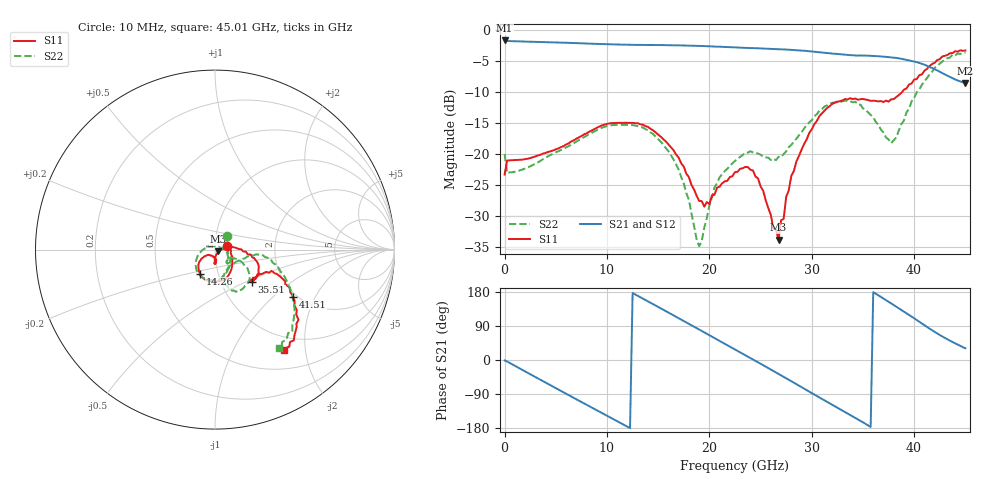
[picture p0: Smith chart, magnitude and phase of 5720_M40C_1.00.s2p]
! Device:  ADRF5720
! Description: 0.5dB LSB GaAs MMIC 6-bit Digital Attenuator
! Frequency:  0.000009 -  40 GHz
! Ports:
!	RF1	= Port 1
!	RF2	= Port 2
! Vdd:  3.3 Volt
! Vss:  -3.3 Volt
! Control:  0/3.3 Volt
! State:  1.00 dB attenuation
! Data:  The device was measured using G-S-G Probes on a matrix board.
!  Data was collected using an calibrated 4 port network analyzer.
!  The reference plane for this measurement is at the launchers.
! Note:  Analog Devices supplies this data as a sample of measured data
!  for this product.  Your particular data for this product may vary.
!  Data was taken at -40 degrees C.
!  Analog Devices reserves the right to change this data at anytime.
# GHZ S DB R 45.0
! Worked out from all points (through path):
!   181 points, 10 MHz to 45.01 GHz, reference 45 ohm
!   highest |S21| = -1.76 dB at 10 MHz (marker M1); lowest = -8.6 dB at 45.01 GHz (marker M2)
!   group delay of S21, straight-line fit = 42.4 ps
!   lowest |S11| = -33.8 dB at 26.76 GHz (marker M3), VSWR 1.04, Z = 46.6 - j0.912 ohm
!   |S11| at or under -10 dB: start of sweep to 38.85 GHz
!   |S22| runs from -34.9 to -3.7 dB; largest |S21 - S12| = 0.0032
!   S11 on the Smith chart (normalised r, x): 10 MHz: 1.14, +0.05; 14.26 GHz: 0.82, -0.23; 35.51 GHz: 1.39, -0.54; 41.51 GHz: 1.92, -1.35; 45.01 GHz: 0.78, -1.62
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0.01  -23.32 18.7  -1.76 -1.1  -1.77 -1.1  -20.03 47.3
0.26  -21.09 -0.6  -1.85 -4.1  -1.86 -4.1  -23.11 -0.5
2.26  -20.78 -14.8  -1.95 -33.8  -1.97 -33.9  -22.19 -17.0
4.26  -19.69 -22.5  -2.05 -63.3  -2.07 -63.3  -20.37 -28.2
7.76  -16.88 -50.4  -2.23 -114.5  -2.25 -114.5  -17.31 -59.1
11.01  -15.02 -83.5  -2.41 -161.6  -2.42 -161.7  -15.32 -94.5
14.26  -15.97 -121.6  -2.49 151.1  -2.51 151.1  -16.56 -134.6
15.26  -17.24 -132.2  -2.50 136.3  -2.52 136.3  -18.04 -148.2
17.01  -20.61 -145.8  -2.55 110.4  -2.57 110.3  -22.54 -175.5
19.01  -27.58 -134.1  -2.64 80.4  -2.66 80.3  -34.85 89.0
20.51  -26.58 -91.8  -2.74 57.9  -2.75 57.8  -25.40 2.0
22.76  -22.88 -88.8  -2.90 24.1  -2.92 24.0  -20.78 -35.7
24.76  -23.95 -91.1  -3.02 -6.0  -3.04 -6.1  -19.96 -48.7
26.76  -33.81 -28.6  -3.17 -36.6  -3.19 -36.8  -20.48 -34.1
28.01  -23.54 8.8  -3.27 -56.0  -3.29 -56.2  -18.56 -25.3
30.26  -15.23 -4.0  -3.57 -91.3  -3.59 -91.4  -13.95 -29.5
33.01  -11.40 -26.0  -4.01 -133.7  -4.03 -133.8  -11.54 -51.8
35.51  -11.34 -41.1  -4.21 -172.7  -4.24 -172.8  -13.33 -71.2
37.76  -11.23 -34.6  -4.48 149.4  -4.51 149.2  -18.29 -51.1
39.76  -8.69 -21.4  -5.06 114.5  -5.08 114.3  -11.55 -6.3
41.51  -5.88 -31.0  -6.03 82.7  -6.05 82.5  -7.19 -23.7
45.01  -3.37 -55.5  -8.58 30.9  -8.61 30.7  -3.72 -57.0
